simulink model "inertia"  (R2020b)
settings: Solver=FixedStepAuto  StartTime=0.0  StopTime=10  FixedStep=0.02  RelTol=1e-3
libraries: sldrtlib x1

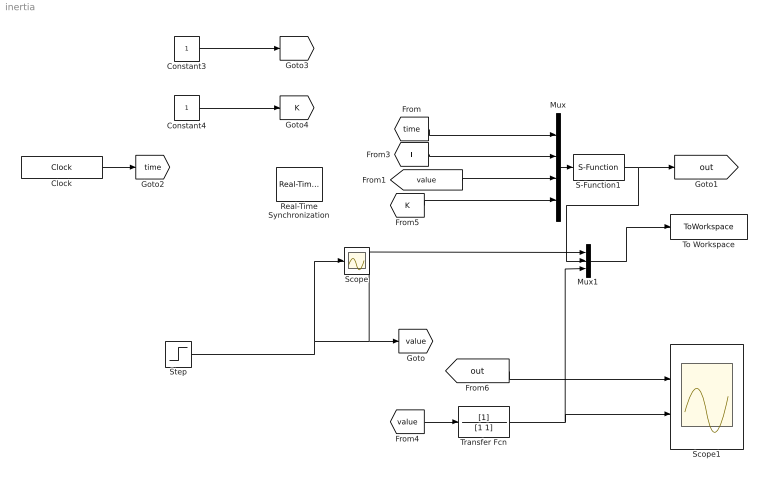
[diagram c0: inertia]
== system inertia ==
  Clock : Clock
  Constant3 : Constant
  Constant4 : Constant
  Mux : Mux
  Mux1 : Mux  Inputs=3
  Real-Time Synchronization : sldrtlib/Real-Time Synchronization  SampleTime=0.02  MaxMissedTicks=inf  ShowMissedTicks=off  YieldWhenWaiting=off
  S-Function1 : S-Function  FunctionName=modbusCominertia  SFunctionDeploymentMode=off  EnableBusSupport=off
  Scope : Scope
  Scope1 : Scope  NumInputPorts=2
  Step : Step  SampleTime=0
  To Workspace : ToWorkspace  VariableName=simout  SampleTime=-1
  Transfer Fcn : TransferFcn  Denominator=[1 1]
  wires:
  S-Function1/1 -> Mux1/2, [out]
  Clock/1 -> [time]
  Transfer Fcn/1 -> Mux1/3, Scope1/2
  [out] -> Scope1/1
  [value] -> Mux/3
  Mux/1 -> S-Function1/1
  [time] -> Mux/1
  [T] -> Mux/2
  Constant3/1 -> [T]
  [value] -> Transfer Fcn/1
  Constant4/1 -> [K]
  [K] -> Mux/4
  Step/1 -> Scope/1, Mux1/1, [value]
  Mux1/1 -> To Workspace/1
